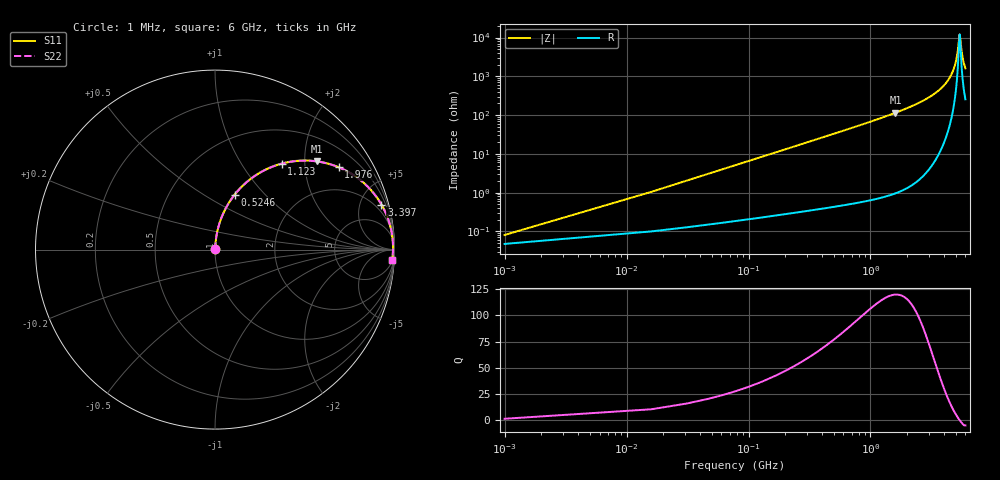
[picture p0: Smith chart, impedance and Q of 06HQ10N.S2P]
! Coilcraft 0604HQ-10N Chip Inductor
! 15 August 2002
# MHZ S MA R 50
!Freq  MagS11  AngS11  MagS21  AngS21  MagS12  AngS12  MagS22  AngS22
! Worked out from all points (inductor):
!   403 points, 1 MHz to 6 GHz, reference 50 ohm
!   read as one part in series: L = 10.4 nH near 30.92 MHz
!   highest Q = 120 at 1.602 GHz (marker M1), where L = 11.4 nH
!   self-resonance near 5.372 GHz
!   S11 on the Smith chart (normalised r, x): 1 MHz: 1.00, +0.00; 524.6 MHz: 1.01, +0.69; 1.123 GHz: 1.01, +1.53; 1.976 GHz: 1.03, +2.98; 3.397 GHz: 1.14, +7.37; 6 GHz: 6, -32
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1  0.0008075 53.9  0.9995 -0.0  0.9995 -0.0  0.0008075 53.9
45.88  0.02996 85.4  0.9981 -1.7  0.9981 -1.7  0.02996 85.4
75.8  0.04942 85.1  0.997 -2.8  0.997 -2.8  0.04942 85.1
105.72  0.06883 84.3  0.9955 -3.9  0.9955 -3.9  0.06883 84.3
165.56  0.1074 82.5  0.9917 -6.2  0.9917 -6.2  0.1074 82.5
255.32  0.1645 79.5  0.9833 -9.5  0.9833 -9.5  0.1645 79.5
524.6  0.3258 70.3  0.9413 -19.0  0.9413 -19.0  0.3258 70.3
1003.32  0.5594 55.4  0.8236 -34.0  0.8236 -34.0  0.5594 55.4
1123  0.6061 52.2  0.79 -37.3  0.79 -37.3  0.6061 52.2
1601.72  0.751 40.8  0.654 -48.7  0.654 -48.7  0.751 40.8
1975.72  0.8274 33.7  0.5546 -55.8  0.5546 -55.8  0.8274 33.7
2005.64  0.8324 33.2  0.547 -56.3  0.547 -56.3  0.8324 33.2
3007.96  0.9398 19.2  0.329 -70.0  0.329 -70.0  0.9398 19.2
3396.92  0.9607 15.1  0.2606 -73.8  0.2606 -73.8  0.9607 15.1
4010.28  0.9805 9.6  0.1668 -78.5  0.1668 -78.5  0.9805 9.6
4608.68  0.9896 5.0  0.08824 -80.7  0.08824 -80.7  0.9896 5.0
5012.6  0.9918 2.3  0.04122 -77.3  0.04122 -77.3  0.9918 2.3
5162.2  0.992 1.4  0.02517 -70.8  0.02517 -70.8  0.992 1.4
5341.72  0.9919 0.3  0.009391 -29.7  0.009391 -29.7  0.9919 0.3
5386.6  0.9918 -0.0  0.008238 0.1  0.008238 0.1  0.9918 -0.0
5670.84  0.9906 -1.7  0.0303 71.2  0.0303 71.2  0.9906 -1.7
6000  0.9884 -3.5  0.06143 77.4  0.06143 77.4  0.9884 -3.5
